FUNCTION "TRASF.CPU" : VOID
TITLE =
AUTHOR : DAVI
VERSION : 0.1

BEGIN
NETWORK
TITLE =
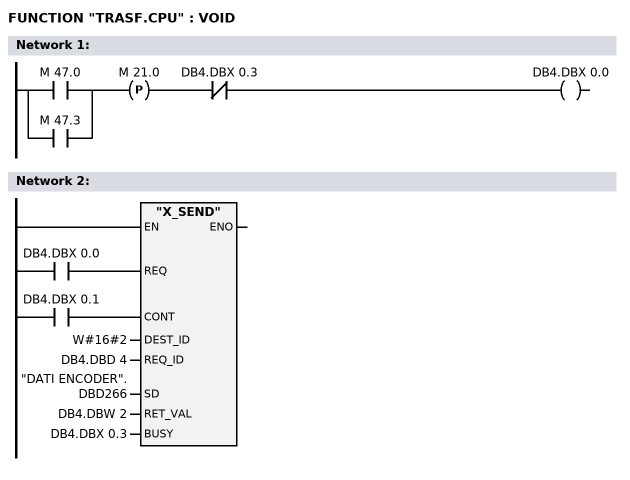
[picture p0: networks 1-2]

      U(    ;
      O     M     47.0;
      O     M     47.3;
      )     ;
      FP    M     21.0;
      UN    DB4.DBX    0.3;
      =     DB4.DBX    0.0;
NETWORK
TITLE =

      U     DB4.DBX    0.0;
      =     L      0.0;
      BLD   103;
      U     DB4.DBX    0.1;
      =     L      0.1;
      BLD   103;
      CALL "X_SEND" (
           REQ                      := L      0.0,
           CONT                     := L      0.1,
           DEST_ID                  := W#16#2,
           REQ_ID                   := DB4.DBD    4,
           SD                       := "DATI ENCODER".DBD266,
           RET_VAL                  := DB4.DBW    2,
           BUSY                     := DB4.DBX    0.3);
      NOP   0;
END_FUNCTION

